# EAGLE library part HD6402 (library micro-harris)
MICROCONTROLLER/MEMORY DEVICE
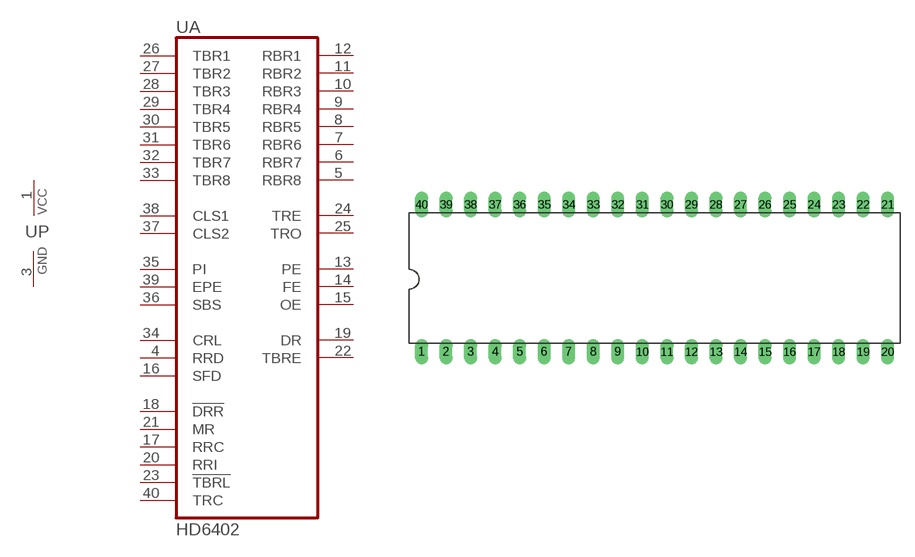
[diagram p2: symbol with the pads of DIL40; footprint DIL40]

Designator prefix U; gates A=HD6402 P=PWRN

## HD6402 (OC_FARNELL: unknown; OC_NEWARK: unknown)  [DIL40]
1  P:VCC  pwr
3  P:GND  pwr
4  A:RRD  in
5  A:RBR8  hiz
6  A:RBR7  hiz
7  A:RBR6  hiz
8  A:RBR5  hiz
9  A:RBR4  hiz
10  A:RBR3  hiz
11  A:RBR2  hiz
12  A:RBR1  hiz
13  A:PE  hiz
14  A:FE  hiz
15  A:OE  hiz
16  A:SFD  in
17  A:RRC  in
18  A:!DRR  in
19  A:DR  hiz
20  A:RRI  in
21  A:MR  in
22  A:TBRE  hiz
23  A:!TBRL  in
24  A:TRE  out
25  A:TRO  out
26  A:TBR1  in
27  A:TBR2  in
28  A:TBR3  in
29  A:TBR4  in
30  A:TBR5  in
31  A:TBR6  in
32  A:TBR7  in
33  A:TBR8  in
34  A:CRL  in
35  A:PI  in
36  A:SBS  in
37  A:CLS2  in
38  A:CLS1  in
39  A:EPE  in
40  A:TRC  in

## Footprint DIL40 (pad centres in mm)
Dual In Line Package
drill 0.813 long: 1 -24.13,-7.62; 2 -21.59,-7.62; 3 -19.05,-7.62; 4 -16.51,-7.62; 5 -13.97,-7.62; 6 -11.43,-7.62; 7 -8.89,-7.62; 8 -6.35,-7.62; 9 -3.81,-7.62; 10 -1.27,-7.62; 11 1.27,-7.62; 12 3.81,-7.62; 13 6.35,-7.62; 14 8.89,-7.62; 15 11.43,-7.62; 16 13.97,-7.62; 17 16.51,-7.62; 18 19.05,-7.62; 19 21.59,-7.62; 20 24.13,-7.62; 21 24.13,7.62; 22 21.59,7.62; 23 19.05,7.62; 24 16.51,7.62; 25 13.97,7.62; 26 11.43,7.62; 27 8.89,7.62; 28 6.35,7.62; 29 3.81,7.62; 30 1.27,7.62; 31 -1.27,7.62; 32 -3.81,7.62; 33 -6.35,7.62; 34 -8.89,7.62; 35 -11.43,7.62; 36 -13.97,7.62; 37 -16.51,7.62; 38 -19.05,7.62; 39 -21.59,7.62; 40 -24.13,7.62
